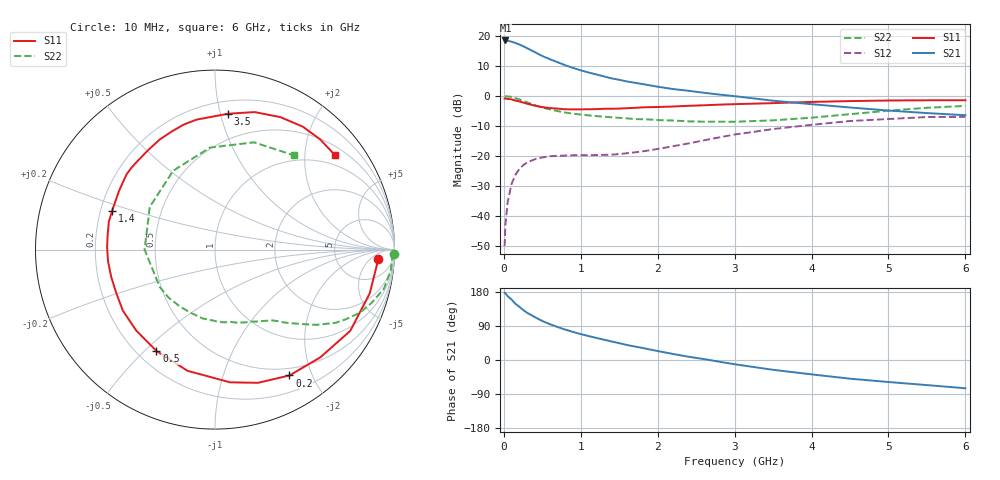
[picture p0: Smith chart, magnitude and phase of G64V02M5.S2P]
! SIEMENS Small Signal Semiconductors
! BFG193
! Si NPN RF Bipolar Junction Transistor in SOT223
! VCE = 4 V  IC = 2.5 mA
! Common Emitter S-Parameters:  August  1996
# GHz  S  MA  R  50
!  f  S11  S21  S12  S22
! GHz  MAG  ANG  MAG  ANG  MAG  ANG  MAG  ANG
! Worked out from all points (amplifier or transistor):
!   36 points, 10 MHz to 6 GHz, reference 50 ohm
!   highest |S21| = 18.6 dB at 20 MHz (marker M1)
!   |S21| within 3 dB of that: start of sweep to 334 MHz
!   unconditionally stable (mu >= 1): 1.32 GHz to 2.55 GHz
!   at 250 MHz: K = 0.20, MSG = 19.9 dB, |S12| = -23.1 dB
!   at 1.4 GHz: K = 1.06, MAG = 11.2 dB, |S12| = -19.6 dB
!   at 6 GHz: K = 0.93, MSG = 0.3 dB, |S12| = -7.0 dB
!   S11 on the Smith chart (normalised r, x): 10 MHz: 16, -10; 200 MHz: 0.40, -1.68; 500 MHz: 0.28, -0.54; 1.4 GHz: 0.25, +0.17; 3.5 GHz: 0.29, +1.06; 6 GHz: 0.71, +2.72
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0.01  0.9115 -3.2  8.414 177.6  0.0031 91.7  0.9958 -1.3
0.02  0.9037 -6.4  8.483 176.4  0.007 88.8  0.9879 -2.7
0.05  0.896 -15.8  8.393 168.4  0.0171 80.9  0.9863 -6.7
0.1  0.8791 -31.0  8.099 159.6  0.0339 74.1  0.9658 -13.1
0.15  0.8394 -45.7  7.706 148.5  0.0483 65.1  0.9207 -18.9
0.2  0.8147 -59.4  7.278 140.6  0.0599 58.7  0.8798 -23.6
0.25  0.7799 -72.1  6.802 132.3  0.0697 52.4  0.8276 -27.9
0.3  0.7443 -83.5  6.321 125.0  0.0774 48.0  0.7857 -31.3
0.4  0.6924 -102.8  5.438 113.5  0.0876 39.8  0.7034 -36.6
0.5  0.6521 -120.0  4.661 102.8  0.0941 33.7  0.6417 -40.3
0.6  0.6294 -134.1  4.122 94.5  0.0986 30.0  0.5969 -43.5
0.7  0.6159 -146.5  3.666 86.9  0.1002 27.2  0.5611 -46.4
0.8  0.6008 -156.6  3.263 80.1  0.1013 25.1  0.5294 -48.8
1.1  0.6014 178.6  2.475 63.2  0.1025 23.6  0.4752 -57.0
1.4  0.6125 159.4  1.972 48.9  0.1048 25.6  0.442 -66.4
1.7  0.6351 144.1  1.668 35.7  0.1145 30.4  0.4126 -77.5
2.2  0.668 123.8  1.307 15.9  0.145 33.6  0.3899 -100.1
2.8  0.7183 104.0  1.058 -4.5  0.2039 29.7  0.372 -133.8
3.5  0.7605 84.5  0.835 -25.9  0.2807 15.6  0.3923 -180.0
4.5  0.8231 63.7  0.643 -49.3  0.3823 -7.7  0.4975 117.9
5.5  0.8486 46.4  0.519 -66.2  0.4459 -36.0  0.636 70.0
6  0.8511 38.2  0.478 -74.6  0.4489 -51.4  0.6844 50.2
